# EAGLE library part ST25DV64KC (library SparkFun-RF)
Dynamic NFC/RFID Dynamic NFC/RFID tag IC with 4-Kbit, 16-Kbit or 64-Kbit EEPROM, fast transfer mode capability and optimized I2C.
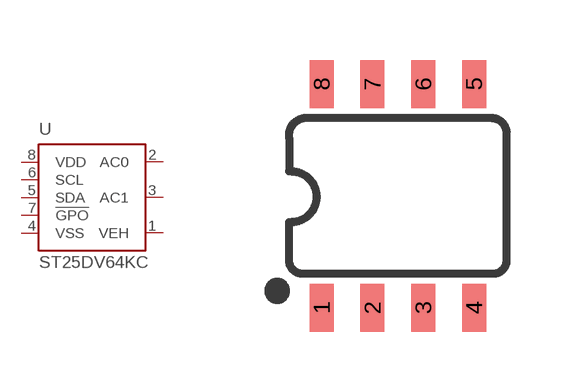
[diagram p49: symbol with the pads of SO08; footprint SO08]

Designator prefix U

## ST25DV64KC (PROD_ID: IC-16315)  [SO08]
1  VEH  pwr
2  AC0
3  AC1
4  VSS  pwr
5  SDA
6  SCL
7  !GPO!  out
8  VDD  pwr

## Footprint SO08 (pad centres in mm)
SOIC, 0.15 inch width
smd 0.6 x 1.2: 1 -1.905,-2.8; 2 -0.635,-2.8; 3 0.635,-2.8; 4 1.905,-2.8; 5 1.905,2.8; 6 0.635,2.8; 7 -0.635,2.8; 8 -1.905,2.8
